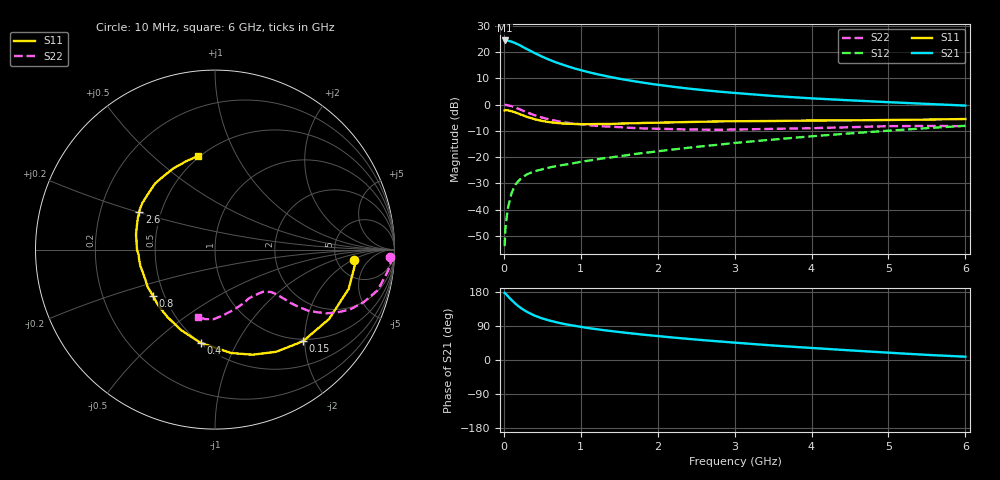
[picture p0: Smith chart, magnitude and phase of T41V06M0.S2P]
! Infineon Technologies  Discrete & RF Semiconductors
! BFR182T
! Si NPN RF Bipolar Junction Transistor in SC75
! VCE = 1 V  IC = 6 mA
! Common Emitter S-Parameters:  October  1999
# GHz  S  MA  R  50
!  f  S11  S21  S12  S22
! GHz  MAG  ANG  MAG  ANG  MAG  ANG  MAG  ANG
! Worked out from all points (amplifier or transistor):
!   36 points, 10 MHz to 6 GHz, reference 50 ohm
!   highest |S21| = 24.4 dB at 10 MHz (marker M1)
!   |S21| within 3 dB of that: start of sweep to 281.6 MHz
!   unconditionally stable (mu >= 1): 1.139 GHz to 4.256 GHz
!   at 250 MHz: K = 0.34, MSG = 24.8 dB, |S12| = -27.6 dB
!   at 1.4 GHz: K = 1.08, MAG = 13.6 dB, |S12| = -20.1 dB
!   at 6 GHz: K = 0.89, MSG = 3.9 dB, |S12| = -8.1 dB
!   S11 on the Smith chart (normalised r, x): 10 MHz: 7.30, -2.20; 150 MHz: 0.96, -1.96; 400 MHz: 0.50, -0.72; 800 MHz: 0.43, -0.28; 2.6 GHz: 0.38, +0.20; 6 GHz: 0.49, +0.71
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0.01  0.777 -4.4  16.68 177.1  0.002 85.6  0.977 -2.3
0.02  0.7864 -5.2  16.68 175.8  0.0043 83.4  0.9875 -2.9
0.05  0.7764 -16.3  16.54 168.8  0.0102 84.3  0.9703 -7.2
0.1  0.7441 -31.3  15.81 158.5  0.0205 77.2  0.9342 -14.0
0.15  0.7078 -46.2  14.79 148.6  0.0297 68.3  0.8775 -19.6
0.2  0.6636 -59.1  13.67 140.4  0.0363 64.2  0.8216 -24.0
0.25  0.622 -70.3  12.48 133.3  0.0417 59.6  0.7623 -27.4
0.3  0.5832 -81.1  11.43 127.1  0.0468 57.1  0.7126 -29.9
0.4  0.5256 -98.8  9.601 117.1  0.0535 52.8  0.6246 -33.2
0.5  0.4866 -112.9  8.171 109.7  0.0585 51.3  0.5644 -34.4
0.6  0.4601 -124.9  7.058 103.7  0.0635 51.2  0.5177 -35.2
0.7  0.4447 -134.9  6.213 98.8  0.0681 51.6  0.4817 -35.4
0.8  0.4314 -143.2  5.541 94.4  0.0718 52.0  0.456 -35.7
1.1  0.4218 -162.9  4.153 84.2  0.0853 54.0  0.4064 -36.6
1.4  0.4267 -176.2  3.321 76.3  0.0985 56.0  0.3786 -38.6
1.6  0.4378 176.3  2.932 71.5  0.1083 57.3  0.3634 -40.0
2.2  0.4578 161.3  2.186 59.3  0.1392 59.6  0.3409 -47.3
2.6  0.4718 153.5  1.882 52.2  0.1614 60.1  0.3324 -53.0
3.5  0.4863 139.0  1.459 38.2  0.2154 59.1  0.3441 -67.2
4.5  0.4995 125.0  1.205 25.4  0.2823 55.4  0.3705 -83.6
5.5  0.5173 108.3  1.03 13.5  0.3555 49.7  0.3911 -97.9
6  0.5308 100.3  0.957 8.7  0.3939 46.0  0.3883 -104.0
